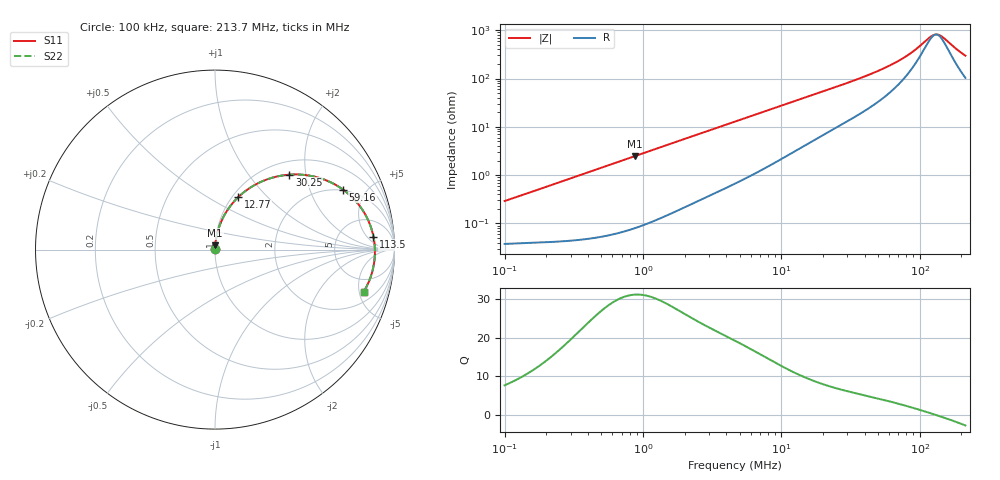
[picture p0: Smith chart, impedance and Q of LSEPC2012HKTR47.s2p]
! LSEPC2012HKTR47  S-PARAMETER MODEL  ( General Type )
! Model Generated by TAIYO YUDEN Corporation (http://www.ty-top.com)
! Version 1.0
! TAIYO YUDEN Control No. 190326NI43SB-FBB
! Copyright(c) 2019 TAIYO YUDEN CO.,LTD. All Rights Reserved.
! Product Description (link to TY-COMPAS)
! https://ds.yuden.co.jp/TYCOMPAS/or/detail?pn=LSEPC2012HKTR47M&u=M
! Products Name : Inductors
! Characteristics :
!  Inductance : 0.47 uH , SRF(min) : -Hz , DC Resistance(max) : 0.035 Ohm
!  Rated Current : Saturation :4100 mA , Temp Rise : 3700 mA (40 degC)
!  Case Size : 2.0 x 1.2 / 0.079 x 0.047 [mm/inch] , Thickness : 0.8 / 0.031 [mm/inch]
!  (Conditions: Temperature = 25 degC , DC Bias Current/Voltage = 0A / 0V)
! External Node Assignments :
!  1  o---GGG---o  2
! GND o---------o GND
! Frequency Range : 0.1MHz  -  213.673535MHz  [ 402 STEP ]
# MHz S RI R 50
! Freq[MHz].  S11 Real  S11 Imag  S21 Real  S21 Imag  S12 Real  S12 Imag  S22 Real  S22 Imag
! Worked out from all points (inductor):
!   401 points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, 100 kHz to 213.7 MHz, reference 50 ohm
!   read as one part in series: L = 456 nH near 103.9 kHz
!   highest Q = 31.1 at 872.3 kHz (marker M1), where L = 451 nH
!   self-resonance near 131.2 MHz
!   S11 on the Smith chart (normalised r, x): 100 kHz: 1.00, +0.01; 12.77 MHz: 1.06, +0.69; 30.25 MHz: 1.26, +1.61; 59.16 MHz: 1.96, +3.45; 113.5 MHz: 12, +8; 213.7 MHz: 3.06, -5.56
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0.1  0.000384 0.00288  0.9996 -0.00288  0.9996 -0.00288  0.000384 0.00288
0.361188  0.000567 0.0103  0.9994 -0.0103  0.9994 -0.0103  0.000567 0.0103
0.872277  0.0014 0.0247  0.9986 -0.0247  0.9986 -0.0247  0.0014 0.0247
1.304567  0.00259 0.0367  0.9974 -0.0367  0.9974 -0.0367  0.00259 0.0367
2.601022  0.00825 0.0718  0.9917 -0.0718  0.9917 -0.0718  0.00825 0.0718
4.71194  0.0231 0.1262  0.9769 -0.1262  0.9769 -0.1262  0.0231 0.1262
8.214983  0.0613 0.2074  0.9387 -0.2074  0.9387 -0.2074  0.0613 0.2074
12.76637  0.1288 0.2916  0.8712 -0.2916  0.8712 -0.2916  0.1288 0.2916
16.69585  0.1948 0.3441  0.8052 -0.3441  0.8052 -0.3441  0.1948 0.3441
30.24575  0.4144 0.4175  0.5856 -0.4175  0.5856 -0.4175  0.4144 0.4175
42.70739  0.5718 0.4021  0.4282 -0.4021  0.4282 -0.4021  0.5718 0.4021
59.15854  0.714 0.334  0.286 -0.334  0.286 -0.334  0.714 0.334
60.30341  0.7216 0.3284  0.2784 -0.3284  0.2784 -0.3284  0.7216 0.3284
71.65743  0.7839 0.2707  0.2161 -0.2707  0.2161 -0.2707  0.7839 0.2707
83.53265  0.8288 0.21  0.1712 -0.21  0.1712 -0.21  0.8288 0.21
95.52717  0.8587 0.1513  0.1413 -0.1513  0.1413 -0.1513  0.8587 0.1513
113.5132  0.8831 0.0705  0.1169 -0.0705  0.1169 -0.0705  0.8831 0.0705
124.9304  0.8895 0.0239  0.1105 -0.0239  0.1105 -0.0239  0.8895 0.0239
137.496  0.8908 -0.0233  0.1092 0.0233  0.1092 0.0233  0.8908 -0.0233
148.4525  0.8881 -0.0612  0.1119 0.0612  0.1119 0.0612  0.8881 -0.0612
190.4603  0.8557 -0.182  0.1443 0.182  0.1443 0.182  0.8557 -0.182
213.6735  0.8286 -0.2346  0.1714 0.2346  0.1714 0.2346  0.8286 -0.2346
